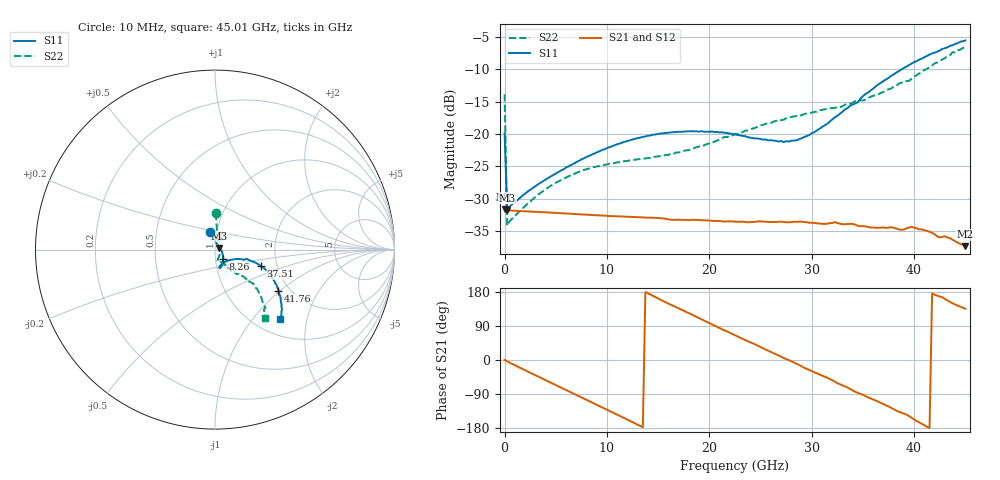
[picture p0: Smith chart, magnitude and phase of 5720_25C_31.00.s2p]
! Device:  ADRF5720
! Description: 0.5dB LSB GaAs MMIC 6-bit Digital Attenuator
! Frequency:  0.000009 -  40 GHz
! Ports:
!	RF1	= Port 1
!	RF2	= Port 2
! Vdd:  3.3 Volt
! Vss:  -3.3 Volt
! Control:  0/3.3 Volt
! State:  31.00 dB attenuation
! Data:  The device was measured using G-S-G Probes on a matrix board.
!  Data was collected using an calibrated 4 port network analyzer.
!  The reference plane for this measurement is at the launchers.
! Note:  Analog Devices supplies this data as a sample of measured data
!  for this product.  Your particular data for this product may vary.
!  Data was taken at 25 degrees C.
!  Analog Devices reserves the right to change this data at anytime.
# GHZ S DB R 45.0
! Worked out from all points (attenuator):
!   181 points, 10 MHz to 45.01 GHz, reference 45 ohm
!   highest |S21| = -31.60 dB at 10 MHz (marker M1); lowest = -37.3 dB at 45.01 GHz (marker M2)
!   lowest |S11| = -31.7 dB at 260 MHz (marker M3), VSWR 1.05, Z = 47.2 + j0.884 ohm
!   |S11| at or under -10 dB: start of sweep to 38.76 GHz
!   |S22| runs from -34.2 to -6.5 dB; largest |S21 - S12| = 0.00018
!   S11 on the Smith chart (normalised r, x): 10 MHz: 0.93, +0.18; 8.26 GHz: 1.09, -0.11; 37.51 GHz: 1.65, -0.33; 41.76 GHz: 1.75, -0.97; 45.01 GHz: 1.30, -1.40
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0.01  -19.87 106.9  -31.60 0.2  -31.60 0.1  -13.85 88.8
0.26  -31.71 21.1  -31.79 -3.7  -31.79 -3.7  -34.16 25.0
1.26  -30.22 2.3  -31.86 -17.1  -31.86 -17.1  -32.25 -7.3
3.51  -27.53 -19.6  -32.04 -46.6  -32.05 -46.6  -29.10 -41.1
5.01  -26.09 -31.1  -32.18 -66.2  -32.18 -66.1  -27.51 -55.3
7.76  -23.72 -46.2  -32.43 -101.9  -32.43 -101.9  -25.55 -69.9
8.26  -23.36 -48.5  -32.48 -108.4  -32.48 -108.4  -25.32 -71.3
12.01  -21.05 -62.0  -32.78 -157.4  -32.78 -157.4  -24.14 -76.4
15.26  -19.90 -69.9  -33.02 158.8  -33.02 158.8  -23.36 -72.4
20.26  -19.58 -75.9  -33.41 93.7  -33.41 93.7  -21.28 -60.2
22.76  -20.13 -75.0  -33.55 62.1  -33.55 62.1  -19.98 -56.3
27.26  -21.23 -56.4  -33.59 5.3  -33.59 5.4  -17.78 -53.4
28.51  -20.96 -46.8  -33.57 -10.0  -33.57 -10.0  -17.20 -54.2
30.26  -19.69 -33.4  -33.73 -32.2  -33.72 -32.1  -16.56 -52.9
34.51  -15.06 -17.4  -34.18 -86.8  -34.19 -86.8  -14.93 -48.5
35.01  -14.11 -17.0  -34.23 -92.1  -34.21 -92.1  -14.80 -47.9
37.51  -11.29 -19.7  -34.46 -122.7  -34.48 -122.5  -13.05 -43.4
37.76  -10.99 -20.4  -34.39 -126.2  -34.38 -126.2  -12.95 -43.1
38.76  -10.00 -22.6  -34.80 -139.0  -34.79 -139.2  -12.04 -43.5
39.76  -9.07 -26.1  -34.36 -152.5  -34.36 -152.6  -11.42 -42.3
41.76  -7.52 -32.9  -35.27 176.1  -35.24 176.1  -9.37 -44.2
45.01  -5.51 -46.6  -37.33 135.3  -37.33 135.2  -6.53 -54.0
